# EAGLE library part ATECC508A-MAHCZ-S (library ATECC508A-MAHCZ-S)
Security ICs / Authentication ICs AWS IOT Provisioned ECC508A 10Kb - 8ld UDFN Generic SWI, 3K T&R Source: Datasheet
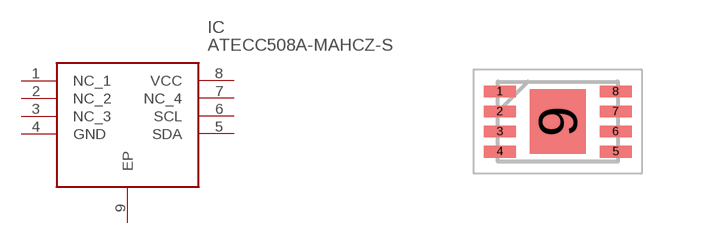
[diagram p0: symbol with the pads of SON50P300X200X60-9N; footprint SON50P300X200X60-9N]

Designator prefix IC

## ATECC508A-MAHCZ-S (Arrow_Part_Number: ATECC508A-MAHCZ-S; Arrow_Price-Stock: https://www.arrow.com/en/products/atecc508a-mahcz-s/microchip-technology?region=nac; Description: Security ICs / Authentication ICs AWS IOT Provisioned ECC508A 10Kb - 8ld UDFN Generic SWI, 3K T&R; Height: 0.6mm; Manufacturer_Name: Microchip; Manufacturer_Part_Number: ATECC508A-MAHCZ-S; Mouser_Part_Number: 556-ATECC508AMAHCZS; Mouser_Price-Stock: https://www.mouser.co.uk/ProductDetail/Microchip-Technology-Atmel/ATECC508A-MAHCZ-S?qs=%2FPOkb%252BiDxRUOydmISUnqmg%3D%3D)  [SON50P300X200X60-9N]
1  NC_1
2  NC_2
3  NC_3
4  GND
5  SDA
6  SCL
7  NC_4
8  VCC
9  EP

## Footprint SON50P300X200X60-9N (pad centres in mm)
8 UDFN
smd 0.8 x 0.3: 1 -1.45,0.75; 2 -1.45,0.25; 3 -1.45,-0.25; 4 -1.45,-0.75; 5 1.45,-0.75; 6 1.45,-0.25; 7 1.45,0.25; 8 1.45,0.75
smd 1.4 x 1.6: 9 0,0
